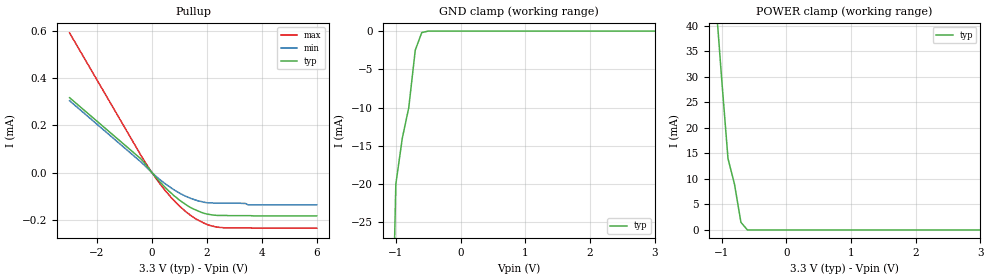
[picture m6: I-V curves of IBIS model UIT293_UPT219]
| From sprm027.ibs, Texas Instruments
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[Model]   UIT293_UPT219
Model_type   Input
Polarity   Non-Inverting
| signals   A, Y
Vinl = 0.8V
Vinh = 2.0V
|   typ   min   max
C_comp   3.5774p   3.4820p   3.7313p
|   typ   min   max
[Temperature Range]   25.0   0   90
|   typ   min   max
[Voltage Range]   3.3V   3.13V   3.47V
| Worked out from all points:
|   slope of the pullup table from 0 to 0.495 V, typ, clamps not added: 7.69 kohm
|   GND clamp passes 1 mA (typ) near -0.63 V on its own axis
|   POWER clamp passes 1 mA (typ) near -0.67 V on its own axis
[GND_clamp]
|   Voltage   I(typ)   I(min)   I(max)
-3V       -900mA     NA         NA
-2V       -400mA     NA         NA
-1V       -20mA      NA         NA
-900mV    -14mA      NA         NA
-800mV    -10mA      NA         NA
-700mV    -2.5mA     NA         NA
-600mV    -200uA     NA         NA
-500mV    0A         NA         NA
3V        0A         NA         NA
[Pullup]
|   Voltage   I(typ)   I(min)   I(max)
-3V       318uA      305uA      593uA
-400mV    58uA       45uA       73uA
-200mV    30uA       23uA       35uA
500mV     -65uA      -49uA      -79uA
800mV     -98uA      -73uA      -118uA
1.2V      -133uA     -99uA      -163uA
1.6V      -159uA     -117uA     -197uA
1.9V      -173uA     -126uA     -215uA
2.4V      -182uA     -130uA     -232uA
3.4V      -183uA     -131uA     -235uA
3.5V      -183uA     -137uA     -235uA
6V        -184uA     -137uA     -236uA
[POWER_clamp]
|   Voltage   I(typ)   I(min)   I(max)
-3V       600mA      NA         NA
-2V       200mA      NA         NA
-1V       30mA       NA         NA
-900mV    14mA       NA         NA
-800mV    9mA        NA         NA
-700mV    1.5mA      NA         NA
-600mV    0A         NA         NA
-500mV    0A         NA         NA
3V        0A         NA         NA
